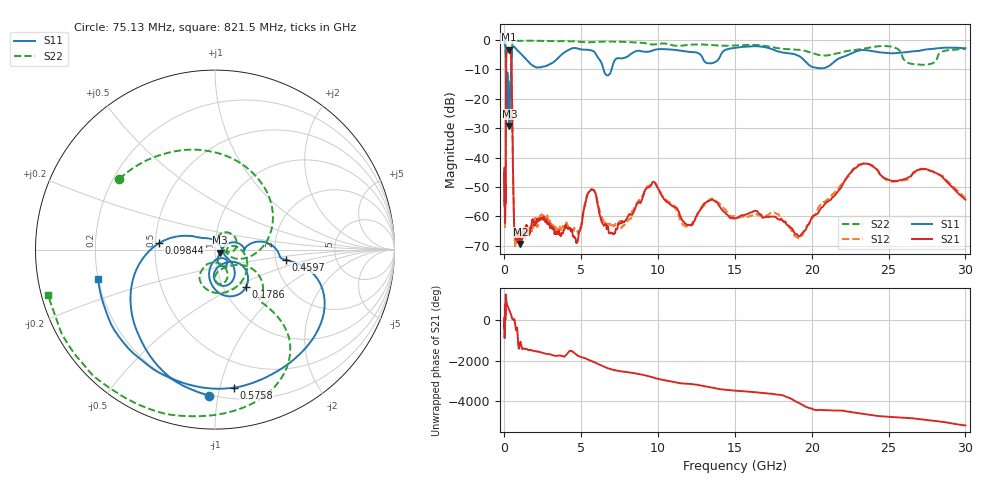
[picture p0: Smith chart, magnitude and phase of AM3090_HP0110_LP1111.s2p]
! Date/Time: Thu, Feb 28, 2019 2:00 PM
! Network Analyzer: Agilent Technologies E8364B Rev: A.07.50.67
! Sweep from 0.010 to 30.000 GHz, 1601 Points, Sweep Type: LOG
! Power Supply: 5.023 V, 0.002 A
# Hz S DB R 50
!freq MagS11 AngS11 MagS21 AngS21 MagS12 AngS12 MagS22 AngS22
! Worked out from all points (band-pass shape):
!   1601 points, 10 MHz to 30 GHz, reference 50 ohm
!   highest |S21| = -3.35 dB at 274.6 MHz (marker M1); lowest = -69.4 dB at 1.034 GHz (marker M2)
!   |S21| within 3 dB of the highest: 113.9 MHz to 442.1 MHz (328.2 MHz wide, 118 % of centre)
!   lowest |S11| = -29.3 dB at 323.9 MHz (marker M3), VSWR 1.07, Z = 53 - j1.89 ohm
!   |S11| at or under -10 dB: 98.41 MHz to 430.2 MHz (331.8 MHz wide, 126 % of centre); 6.447 GHz to 6.976 GHz (528.9 MHz wide, 7.88 % of centre)
!   |S22| runs from -29.3 to -0.2 dB; largest |S21 - S12| = 0.011
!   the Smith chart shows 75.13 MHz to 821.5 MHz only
!   S11 on the Smith chart (normalised r, x): 75.13 MHz: 0.19, -0.94; 98.44 MHz: 0.52, +0.04; 178.6 MHz: 1.27, -0.58; 459.7 MHz: 2.29, -0.32; 575.8 MHz: 0.29, -1.11; 821.5 MHz: 0.20, -0.12
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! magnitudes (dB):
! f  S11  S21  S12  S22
! 10 MHz  -0.3  -45.4  -43.8  -0.7
! 38.04 MHz  -0.5  -60.4  -63.1  -1.7
! 75.13 MHz  -1.8  -54.3  -52.7  -3.6
! 98.44 MHz  -10.0  -18.6  -18.5  -11.1
! 107.2 MHz  -28.6  -8.5  -8.5  -28.7
! 144.7 MHz  -20.8  -4.0  -4.0  -23.3
! 178.6 MHz  -11.3  -3.6  -3.6  -13.7
! 274.6 MHz  -19.9  -3.3  -3.3  -19.5
! 323.9 MHz  -29.3  -3.5  -3.5  -19.3
! 459.7 MHz  -7.9  -8.5  -8.4  -7.7
! 550.5 MHz  -2.3  -42.6  -42.6  -0.5
! 575.8 MHz  -2.2  -50.2  -50.3  -0.4
! 821.5 MHz  -3.5  -64.8  -67.6  -0.3
! 1.034 GHz  -4.6  -69.4  -66.9  -0.3
! 2.084 GHz  -9.4  -62.1  -62.4  -0.3
! 4.64 GHz  -2.8  -67.7  -64.4  -0.5
! 5.668 GHz  -3.6  -50.8  -50.9  -0.8
! 7.926 GHz  -5.9  -61.0  -62.0  -0.7
! 9.538 GHz  -3.9  -49.6  -49.3  -1.6
! 19.03 GHz  -5.2  -66.0  -66.9  -3.4
! 23.24 GHz  -3.5  -42.2  -42.4  -3.1
! 30 GHz  -2.8  -54.3  -53.6  -3.1
